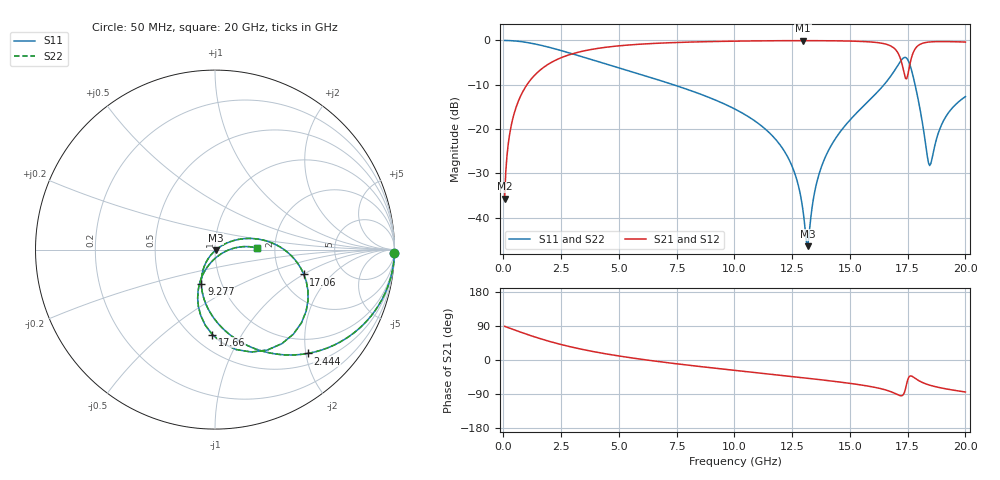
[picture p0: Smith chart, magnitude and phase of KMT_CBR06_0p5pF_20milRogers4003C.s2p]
! Data measured by Modelithics Inc. support@modelithics.com 813-866-6335
! KEMET CBR0603 0.5pF, Pad Width= 0.851mm, Pad Length= 0.64mm, Pad Gap= 0.62mm, 20mil Rogers 4003C substrate Data, January 2022
# hz S ma R 50
! 2 Port Network Data from SP1.SP block
! freq  magS11  angS11  magS21  angS21  magS12  angS12  magS22  angS22
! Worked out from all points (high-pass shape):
!   401 points, 50 MHz to 20 GHz, reference 50 ohm
!   highest |S21| = -0.04 dB at 12.97 GHz (marker M1); lowest = -35.7 dB at 50 MHz (marker M2)
!   |S21| within 3 dB of the highest: 2.968 GHz to 17.1 GHz (14.13 GHz wide, 141 % of centre); 17.72 GHz to end of sweep
!   lowest |S11| = -46.5 dB at 13.17 GHz (marker M3), VSWR 1.01, Z = 50.3 - j0.325 ohm
!   |S11| at or under -10 dB: 7.356 GHz to 16.48 GHz (9.12 GHz wide, 76.5 % of centre); 17.82 GHz to end of sweep
!   |S22| runs from -46.5 to 0.0 dB; largest |S21 - S12| = 0
!   S11 on the Smith chart (normalised r, x): 50 MHz: open; 2.444 GHz: 0.70, -2.04; 9.277 GHz: 0.80, -0.32; 17.06 GHz: 2.68, -1.01; 17.66 GHz: 0.62, -0.76; 20 GHz: 1.60, +0.03
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5e7  0.9999 -1.1  0.01632 88.9  0.01632 88.9  0.9999 -1.1
2.99375e8  0.9952 -6.7  0.0973 83.3  0.0973 83.3  0.9952 -6.7
6.98375e8  0.9748 -15.5  0.2226 74.5  0.2226 74.5  0.9748 -15.5
2.444e9  0.7756 -48.2  0.6298 41.7  0.6298 41.7  0.7756 -48.2
3.391625e9  0.6564 -61.6  0.7526 28.3  0.7526 28.3  0.6564 -61.6
6.73325e9  0.3565 -93.8  0.9315 -4.3  0.9315 -4.3  0.3565 -93.8
9.276875e9  0.2069 -111.5  0.9748 -22.4  0.9748 -22.4  0.2069 -111.5
1.0025e10  0.1677 -116.2  0.9821 -27.4  0.9821 -27.4  0.1677 -116.2
1.211975e10  0.05842 -127.1  0.9938 -41.1  0.9938 -41.1  0.05842 -127.1
1.266838e10  0.02849 -125.9  0.9948 -44.8  0.9948 -44.8  0.02849 -125.9
1.296762e10  0.01207 -114.4  0.9949 -46.8  0.9949 -46.8  0.01207 -114.4
1.316712e10  0.004747 -42.9  0.9948 -48.1  0.9948 -48.1  0.004747 -42.9
1.336662e10  0.01323 18.8  0.9946 -49.5  0.9946 -49.5  0.01323 18.8
1.366588e10  0.03107 28.9  0.9939 -51.6  0.9939 -51.6  0.03107 28.9
1.42145e10  0.06679 29.5  0.9915 -55.6  0.9915 -55.6  0.06679 29.5
1.670825e10  0.3765 0.9  0.8812 -82.1  0.8812 -82.1  0.3765 0.9
1.705738e10  0.5143 -15.6  0.7386 -91.2  0.7386 -91.2  0.5143 -15.6
1.74065e10  0.6429 -54.6  0.3731 -76.2  0.3731 -76.2  0.6429 -54.6
1.765588e10  0.4743 -91.7  0.6244 -42.2  0.6244 -42.2  0.4743 -91.7
1.845388e10  0.03863 -55.1  0.9615 -66.4  0.9615 -66.4  0.03863 -55.1
1.910225e10  0.1309 5.9  0.9715 -75.5  0.9715 -75.5  0.1309 5.9
2e10  0.2322 2.4  0.9594 -84.4  0.9594 -84.4  0.2322 2.4
